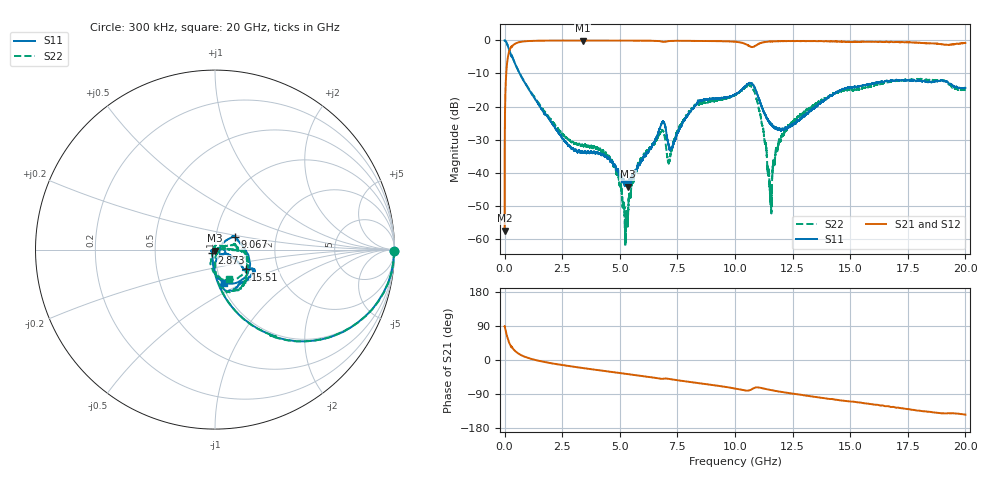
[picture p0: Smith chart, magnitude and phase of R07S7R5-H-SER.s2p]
!{R07S7R5}
!Johanson Technology Inc.
!www.johansontechnology.com
!Test Board Conditions:
!Substrate Type  RO4350B
!Substrate Thickness  10 mil
!Substrate Dk  3.66
!TL Type: GCPW
!TL Trace Width  21 mil
!TL Gap  20 mil
!Electrode orientation  Horizontal
!DUT TOPOLOGY	SERIES
!Mounting Pad LxW  16x21 mil
! Created Sat Feb  6 11:39:36 2021
# hz S ma R 50
! 2 Port Network Data from SP1.SP block
! freq  magS11  angS11  magS21  angS21  magS12  angS12  magS22  angS22
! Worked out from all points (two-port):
!   20001 points, 300 kHz to 20 GHz, reference 50 ohm
!   highest |S21| = -0.02 dB at 3.386 GHz (marker M1); lowest = -57.6 dB at 300 kHz (marker M2)
!   |S21| within 3 dB of the highest: 210.6 MHz to end of sweep
!   lowest |S11| = -44.3 dB at 5.357 GHz (marker M3), VSWR 1.01, Z = 50 - j0.608 ohm
!   |S11| at or under -10 dB: 654 MHz to end of sweep
!   |S22| runs from -62.3 to 0.0 dB; largest |S21 - S12| = 0.014
!   S11 on the Smith chart (normalised r, x): 300 kHz: open; 2.873 GHz: 0.97, -0.03; 9.067 GHz: 1.23, +0.18; 15.51 GHz: 1.37, -0.32; 20 GHz: 1.03, -0.40
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300000  0.9982 -0.4  0.001322 89.4  0.001527 90.2  0.9983 -0.4
1.083e8  0.8873 -27.9  0.4564 62.4  0.4568 62.4  0.888 -27.8
2.733e8  0.6043 -54.5  0.7894 36.1  0.7899 36.0  0.6064 -54.6
8.853e8  0.2262 -81.6  0.9714 8.3  0.971 8.3  0.2293 -80.9
2.8733e9  0.0236 -134.0  0.9969 -16.7  0.9957 -16.7  0.02957 -73.7
3.3343e9  0.02064 -154.5  0.9963 -20.7  0.996 -20.7  0.02594 -63.5
3.3863e9  0.02056 -157.1  0.9972 -21.1  0.9962 -21.2  0.02612 -60.4
4.5923e9  0.01486 -161.4  0.9953 -31.1  0.9956 -31.1  0.01486 -64.2
5.3573e9  0.006091 -86.0  0.9937 -37.2  0.9941 -37.3  0.002381 125.8
5.7293e9  0.01103 -39.8  0.9932 -40.2  0.9929 -40.3  0.01066 109.4
6.6673e9  0.03972 4.6  0.9822 -48.4  0.9822 -48.4  0.0356 47.3
7.1403e9  0.02409 -26.8  0.9789 -49.9  0.978 -49.9  0.01391 7.1
7.9323e9  0.07227 40.2  0.9857 -57.0  0.9863 -57.0  0.07399 16.7
9.0673e9  0.1312 33.2  0.9786 -66.5  0.979 -66.5  0.1207 7.8
1.00003e10  0.1518 9.1  0.9563 -75.3  0.957 -75.4  0.1484 0.5
1.08203e10  0.2035 -68.3  0.8063 -74.1  0.8082 -74.2  0.1749 -74.0
1.15233e10  0.05658 -78.0  0.9643 -78.9  0.964 -78.9  0.005932 -34.6
1.19823e10  0.04421 -52.3  0.9761 -83.9  0.9756 -83.9  0.03095 12.2
1.33343e10  0.08874 -19.6  0.9778 -96.0  0.978 -96.0  0.0992 -1.8
1.55143e10  0.2043 -32.8  0.9611 -113.3  0.9573 -113.1  0.188 -18.6
1.66673e10  0.2395 -27.0  0.9407 -122.2  0.9449 -122.7  0.2339 -41.8
2e10  0.1916 -74.2  0.9178 -144.3  0.9135 -144.3  0.1823 -64.8
